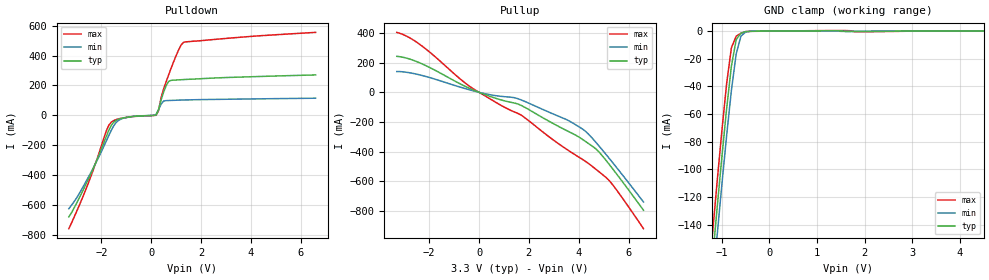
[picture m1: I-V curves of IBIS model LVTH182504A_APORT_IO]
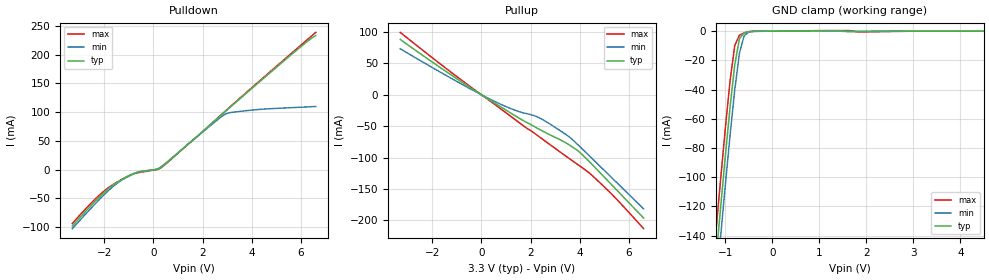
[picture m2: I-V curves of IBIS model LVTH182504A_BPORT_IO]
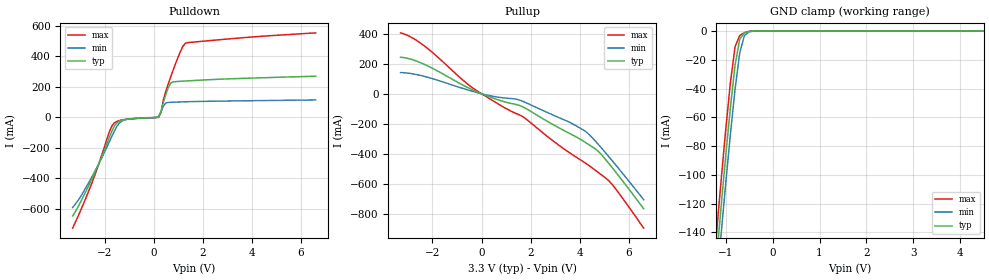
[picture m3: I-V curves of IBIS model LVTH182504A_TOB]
|   TEXAS INSTRUMENTS INCORPORATED
|   Standard Linear and Logic
|   IBIS Model of SN74LVTH182504A
|   3.3V ABT SCAN TEST DEVICES WITH 20-BIT UNIVERSAL BUS TRANSCEIVERS
[IBIS Ver]   2.1
[Comment char]   |_char
[File Name]   sn74lvth182504a.ibs
[File Rev]   1.2   | from silicon model only
[Date]   01/31/2001
[Source]   Silicon-level SPICE model at Texas Instruments (ALEY)
[Notes]
   3.3-V ABT SCAN TEST DEVICES WITH 20-BIT UNIVERSAL BUS TRANSCEIVERS
   !! SN74LVTH182504A is available and preferred vs SN74LVT182504 !!
   Release 1.0) 97104 ALEY
   Release 1.1) 97212 ALEY (based on process model updates)
   Release 1.2) 97215 ALEY - fixed load for ramp (rising) measurement
   includes all available commercial packages:
   PM=64TQFP (no-coupling model)
   - This file may be incomplete or may not be fully compliant
   with the IBIS specification. It will be replaced with a
   version that is IBIS Revision 3.2 compliant and is complete
   and accurate. Please email all questions and comments to
   sllibis@ti.com.
|   -For Questions or Comments please mailto:sllibis@ti.com
|  [Disclaimer]
|*   Property of Texas Instruments Incorporated.  Unauthorized   *
|*   reproduction and/or distribution is strictly prohibited.   *
|*   This product is protected under copyright law.   *
|*   Created 1995, (C) Copyright 1995, Texas Instruments Inc.,   *
|*   All Rights Reserved   *
|*   UNLESS THERE IS A SIGNED, WRITTEN AGREEMENT TO THE   *
|*   CONTRARY, TEXAS INSTRUMENTS ("TI") IS PROVIDING THE SPICE   *
|*   MODELS "AS IS" AND WITHOUT ANY WARRANTY, EXPRESSED OR   *
|*   IMPLIED.  TI assumes no liability for:   *
|*   1) the accuracy of the IBIS models provided to your   *
|*   company;   *
|*   2) the proper functioning of these IBIS models in your   *
|*   design or for any resulting applications; or   *
|*   3) infringement of patents, copyrights or intellectual   *
|*   property rights resulting from your use of these   *
|*   IBIS models.   *
|*   TI provides IBIS Models as a service to our customers.   *
|*   You and your company shall not distribute, sell or give   *
|*   these models to anyone else without prior written   *
|*   permission from TI.   *
|*   TI reserves the right to make changes to our products or   *
|*   to discontinue any semiconductor product or service   *
|*   without notice, and advises our customers to obtain the   *
|*   latest version of relevant information to verify, before   *
|*   placing orders, that the information being relied on is   *
|*   current.   *
|*   Please be aware that your receipt and use of the IBIS   *
|*   information provided shall serve as acceptance of these   *
|*   terms and conditions.  If you do not accept these terms,   *
|*   you should return or destroy the IBIS models and any   *
|*   other accompanying information immediately.   *
[Component]   SN74LVTH182504APM
[Manufacturer]  Texas Instruments
[Package]
|   typ   min   max
R_pkg   0.03   0.027   0.034
L_pkg   2.066nH   1.969nH   2.225nH
C_pkg   0.104pF   0.075pF   0.188pF
[Pin]   signal_name  model_name   R_pin   L_pin   C_pin
1   A4   LVTH182504A_APORT_IO   0.03   2.212nH   0.188pF
2   A5   LVTH182504A_APORT_IO   0.029   2.132nH   0.114pF
3   A6   LVTH182504A_APORT_IO   0.03   2.093nH   0.099pF
4   GND   GND   0.03   2.08nH   0.106pF
5   A7   LVTH182504A_APORT_IO   0.032   2.05nH   0.087pF
6   A8   LVTH182504A_APORT_IO   0.032   2.015nH   0.08pF
7   A9   LVTH182504A_APORT_IO   0.033   2.007nH   0.077pF
8   A10   LVTH182504A_APORT_IO   0.032   1.99nH   0.08pF
9   VCC   POWER   0.033   2.074nH   0.09pF
10   A11   LVTH182504A_APORT_IO   0.032   1.995nH   0.075pF
11   A12   LVTH182504A_APORT_IO   0.032   2.025nH   0.08pF
12   A13   LVTH182504A_APORT_IO   0.031   2.033nH   0.085pF
13   GND   GND   0.03   2.093nH   0.105pF
14   A14   LVTH182504A_APORT_IO   0.031   2.142nH   0.1pF
15   A15   LVTH182504A_APORT_IO   0.03   2.166nH   0.114pF
16   A16   LVTH182504A_APORT_IO   0.029   2.225nH   0.188pF
17   A17   LVTH182504A_APORT_IO   0.03   2.213nH   0.188pF
18   A18   LVTH182504A_APORT_IO   0.031   2.161nH   0.114pF
19   A19   LVTH182504A_APORT_IO   0.032   2.142nH   0.1pF
20   GND   GND   0.031   2.106nH   0.105pF
21   A20   LVTH182504A_APORT_IO   0.032   2.054nH   0.085pF
22   NCLKENAB  LVTH182504A_INC   0.032   2.017nH   0.077pF
23   CLKAB   LVTH182504A_INC   0.033   2.065nH   0.079pF
24   TDI   LVTH182504A_INU   0.034   2.087nH   0.084pF
25   VCC   POWER   0.032   2.049nH   0.086pF
26   TCK   LVTH182504A_INT   0.032   1.989nH   0.075pF
27   LEAB   LVTH182504A_INC   0.032   2.014nH   0.079pF
28   NOEAB   LVTH182504A_INU   0.032   2.049nH   0.086pF
29   GND   GND   0.03   2.073nH   0.105pF
30   B20   LVTH182504A_BPORT_IO   0.03   2.097nH   0.099pF
31   B19   LVTH182504A_BPORT_IO   0.031   2.142nH   0.114pF
32   B18   LVTH182504A_BPORT_IO   0.028   2.178nH   0.187pF
33   B17   LVTH182504A_BPORT_IO   0.028   2.167nH   0.187pF
34   B16   LVTH182504A_BPORT_IO   0.027   2.082nH   0.112pF
35   B15   LVTH182504A_BPORT_IO   0.029   2.08nH   0.099pF
36   GND   GND   0.029   2.064nH   0.105pF
37   B14   LVTH182504A_BPORT_IO   0.029   2.008nH   0.085pF
38   B13   LVTH182504A_BPORT_IO   0.03   1.98nH   0.079pF
39   B12   LVTH182504A_BPORT_IO   0.031   1.981nH   0.077pF
40   B11   LVTH182504A_BPORT_IO   0.031   1.976nH   0.08pF
41   VCC   POWER   0.033   2.005nH   0.081pF
42   B10   LVTH182504A_BPORT_IO   0.031   1.97nH   0.076pF
43   B9   LVTH182504A_BPORT_IO   0.031   1.996nH   0.08pF
44   B8   LVTH182504A_BPORT_IO   0.031   2.03nH   0.086pF
45   GND   GND   0.03   2.072nH   0.105pF
46   B7   LVTH182504A_BPORT_IO   0.03   2.102nH   0.1pF
47   B6   LVTH182504A_BPORT_IO   0.029   2.11nH   0.113pF
48   B5   LVTH182504A_BPORT_IO   0.028   2.155nH   0.186pF
49   B4   LVTH182504A_BPORT_IO   0.028   2.157nH   0.186pF
50   B3   LVTH182504A_BPORT_IO   0.028   2.09nH   0.112pF
51   B2   LVTH182504A_BPORT_IO   0.028   2.078nH   0.099pF
52   GND   GND   0.029   2.047nH   0.105pF
53   B1   LVTH182504A_BPORT_IO   0.028   1.996nH   0.085pF
54   NCLKENBA  LVTH182504A_INC   0.029   1.969nH   0.079pF
55   CLKBA   LVTH182504A_INC   0.031   1.97nH   0.077pF
56   TMS   LVTH182504A_INU   0.031   1.975nH   0.08pF
57   VCC   POWER   0.032   1.985nH   0.08pF
58   TDO   LVTH182504A_TOB   0.031   1.98nH   0.077pF
59   LEBA   LVTH182504A_INC   0.03   1.987nH   0.08pF
60   NOEBA   LVTH182504A_INU   0.03   2.022nH   0.086pF
61   GND   GND   0.029   2.068nH   0.105pF
62   A1   LVTH182504A_APORT_IO   0.03   2.086nH   0.099pF
63   A2   LVTH182504A_APORT_IO   0.029   2.117nH   0.113pF
64   A3   LVTH182504A_APORT_IO   0.029   2.167nH   0.186pF
| Models and submodels in the file (6): LVTH182504A_APORT_IO (I/O), LVTH182504A_BPORT_IO (I/O), LVTH182504A_TOB (3-state), LVTH182504A_INC (Input), LVTH182504A_INT (Input), LVTH182504A_INU (Input)
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[Model]   LVTH182504A_APORT_IO
| high-drive I/O buffer with bus-hold
| ibuf.lvta (97212 ALEY)
| tob.lvta  (97212 ALEY)
| pad.lvta  (97212 ALEY)
| Signals   A1..A20
Model_type  I/O
Polarity   Non-Inverting
Enable   Active-Low
Vinl = 0.8V
Vinh = 2.0V
Vmeas= 1.5V
Cref = 50pf
Rref = 500
Vref = 0V
| variable   typ   min   max
C_comp   10p   NA   NA
[Temperature Range]   50   100   0
[Voltage range]   3.3   3   3.6
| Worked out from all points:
|   slope of the pulldown table from 0 to 0.495 V, typ, clamps not added: 3.25 ohm
|   slope of the pullup table from 0 to 0.495 V, typ, clamps not added: 16.2 ohm
|   GND clamp passes 1 mA (typ) near -0.56 V on its own axis
|Process range|   weak   strong
[pullup]
|   50C:3.3V:   100C:3V:weak   0C:3.6V:strong
|   Voltage   I(typ)   I(min)   I(max)
-3.3V     242.7mA    140.2mA    404.2mA
-2.8V     225.4mA    132.2mA    369.3mA
-2.3V     192.9mA    114.1mA    313.8mA
-300mV    20.86mA    13.18mA    31.49mA
700mV     -41.94mA   -23.2mA    -70.26mA
1.5V      -75.64mA   -39.93mA   -138.1mA
1.8V      -97.86mA   -58.74mA   -166.6mA
3.6V      -265.2mA   -191.6mA   -393.7mA
4.3V      -334.7mA   -267.1mA   -469.1mA
4.7V      -383.4mA   -339.3mA   -520.3mA
5.2V      -480.9mA   -440.4mA   -590.8mA
6.6V      -795.3mA   -739.8mA   -919.7mA
[pulldown]
|   50C:3.3V:   100C:3V:weak   0C:3.6V:strong
|   Voltage   I(typ)   I(min)   I(max)
-3.3V     -677.8mA   -623.8mA   -757mA
-2.5V     -420.1mA   -407.9mA   -444.4mA
-1.8V     -141.6mA   -172.1mA   -104.6mA
-1.6V     -67.02mA   -100.3mA   -45.51mA
-1.4V     -32.5mA    -46.74mA   -27.93mA
200mV     2.567mA    6.67mA     823.3uA
300mV     39.57mA    39.07mA    32.13mA
500mV     154.4mA    95.69mA    175mA
700mV     226.4mA    99.55mA    269.2mA
1.1V      237.5mA    101.9mA    436.1mA
1.3V      239.4mA    103mA      488.3mA
6.6V      270.5mA    114.9mA    554.8mA
[gnd_clamp]
|   50C:3.3V:   100C:3V:weak   0C:3.6V:strong
|   Voltage   I(typ)   I(min)   I(max)
-3.3V     -1.549A    -1.512A    -1.612A
-1.2V     -166.4mA   -186.3mA   -147.8mA
-1.1V     -128.1mA   -148mA     -109.1mA
-1V       -91.01mA   -111mA     -72.06mA
-900mV    -56mA      -75.56mA   -37.94mA
-800mV    -25.34mA   -42.9mA    -12mA
-700mV    -6.279mA   -16.54mA   -3.704mA
-600mV    -1.455mA   -3.641mA   -1.512mA
-500mV    -329uA     -657.6uA   -358.3uA
-300mV    -77.95uA   -53.31uA   -119.1uA
1.4V      233.8uA    101uA      404.8uA
6.6V      11.17nA    12.21nA    10.92nA
[ramp]
| variable   typ   min   max
dV/dt_r   1.5089E+00/4.8115E-10  1.1420E+00/1.4491E-09  1.7783E+00/2.2391E-10
dV/dt_f   1.7910E+00/8.5545E-10  1.6177E+00/2.2914E-09  1.9765E+00/4.1736E-10
[Model]   LVTH182504A_BPORT_IO
| high-drive I/O buffer with bus-hold
| ibuf.lvta (97212 ALEY)
| t25.lvta  (97212 ALEY)
| pad.lvta  (97212 ALEY)
| Signals   B1..B20
Model_type  I/O
Polarity   Non-Inverting
Enable   Active-Low
Vinl = 0.8V
Vinh = 2.0V
Vmeas= 1.5V
Cref = 50pf
Rref = 500
Vref = 0V
| variable   typ   min   max
C_comp   10p   NA   NA
[Temperature Range]   50   100   0
[Voltage range]   3.3   3   3.6
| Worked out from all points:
|   slope of the pulldown table from 0 to 0.495 V, typ, clamps not added: 45.3 ohm
|   slope of the pullup table from 0 to 0.495 V, typ, clamps not added: 40.7 ohm
|   GND clamp passes 1 mA (typ) near -0.58 V on its own axis
|Process range|   weak   strong
[pullup]
|   50C:3.3V:   100C:3V:weak   0C:3.6V:strong
|   Voltage   I(typ)   I(min)   I(max)
-3.3V     87.93mA    73.1mA     99.21mA
-1.6V     41.29mA    34.42mA    46.83mA
200mV     -4.944mA   -4.077mA   -5.666mA
1.3V      -31.73mA   -23.61mA   -37.44mA
2.3V      -53.86mA   -35.71mA   -65.38mA
3.2V      -71.57mA   -57.06mA   -91.07mA
3.6V      -80.55mA   -67.91mA   -102.3mA
3.9V      -88.5mA    -78.65mA   -110.6mA
4.5V      -110.9mA   -101.4mA   -128.3mA
5.4V      -147.4mA   -135.8mA   -162.2mA
6.6V      -196.3mA   -181.6mA   -213.2mA
[pulldown]
|   50C:3.3V:   100C:3V:weak   0C:3.6V:strong
|   Voltage   I(typ)   I(min)   I(max)
-3.3V     -98.29mA   -102.9mA   -93.91mA
-2.3V     -52.13mA   -56.52mA   -48.52mA
-1.9V     -35.93mA   -39.45mA   -33.8mA
-1.5V     -22.87mA   -24.62mA   -22.42mA
-700mV    -5.307mA   -5.472mA   -6.239mA
100mV     25.12uA    283.8uA    -376.2uA
300mV     3.666mA    4.577mA    2.833mA
2.9V      100.2mA    95.86mA    100.8mA
3.1V      107.6mA    98.94mA    108.5mA
4.2V      148.5mA    104.2mA    149.9mA
6V        214mA      108.5mA    216.5mA
6.6V      233.1mA    109.7mA    238.6mA
[gnd_clamp]
|   50C:3.3V:   100C:3V:weak   0C:3.6V:strong
|   Voltage   I(typ)   I(min)   I(max)
-3.3V     -969.6mA   -991mA     -949.1mA
-1.2V     -156.2mA   -176mA     -137mA
-1.1V     -120.2mA   -140.1mA   -101mA
-1V       -85.23mA   -105mA     -66.15mA
-900mV    -52mA      -71.24mA   -33.96mA
-800mV    -22.87mA   -40.05mA   -9.759mA
-700mV    -5.117mA   -14.95mA   -2.748mA
-600mV    -1.165mA   -3.046mA   -1.228mA
-500mV    -309.2uA   -581.3uA   -349.3uA
-300mV    -77.95uA   -53.3uA    -119.1uA
1.4V      233.8uA    101uA      404.8uA
6.6V      11.17nA    12.21nA    10.92nA
[ramp]
| variable   typ   min   max
dV/dt_r   1.0791E+00/4.8409E-10  8.6453E-01/1.4920E-09  1.2563E+00/2.4887E-10
dV/dt_f   1.2133E+00/7.4384E-10  1.1004E+00/1.8193E-09  1.3392E+00/3.7318E-10
[Model]   LVTH182504A_TOB
| three-state output buffer
| tob.lvta (97212 ALEY)
| pad.lvta (97212 ALEY)
| Signals   TDO
Model_type  3-state
Polarity   Non-Inverting
Enable   Active-Low
Vinl = 0.8V
Vinh = 2.0V
Vmeas= 1.5V
Cref = 50pf
Rref = 500
Vref = 0V
| variable   typ   min   max
C_comp   8p   NA   NA
[Temperature Range]   50   100   0
[Voltage range]   3.3   3   3.6
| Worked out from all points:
|   slope of the pulldown table from 0 to 0.495 V, typ, clamps not added: 3.25 ohm
|   slope of the pullup table from 0 to 0.495 V, typ, clamps not added: 16.2 ohm
|   GND clamp passes 1 mA (typ) near -0.58 V on its own axis
|Process range|   weak   strong
[pullup]
|   50C:3.3V:   100C:3V:weak   0C:3.6V:strong
|   Voltage   I(typ)   I(min)   I(max)
-3.3V     242.7mA    140.2mA    404.2mA
-2.8V     225.4mA    132.2mA    369.3mA
-2.3V     192.9mA    114.1mA    313.8mA
-300mV    20.86mA    13.18mA    31.49mA
700mV     -41.88mA   -23.15mA   -70.19mA
1.5V      -75.36mA   -39.76mA   -137.7mA
1.8V      -97.58mA   -58.87mA   -166.1mA
3.6V      -265.1mA   -191mA     -393.7mA
4.3V      -331mA     -259mA     -468.4mA
4.7V      -375mA     -326.3mA   -516.3mA
5.2V      -466.4mA   -421.4mA   -580.8mA
6.6V      -763.6mA   -703.5mA   -892.5mA
[pulldown]
|   50C:3.3V:   100C:3V:weak   0C:3.6V:strong
|   Voltage   I(typ)   I(min)   I(max)
-3.3V     -646.1mA   -591.2mA   -726.1mA
-2.5V     -398.2mA   -385.2mA   -423.3mA
-1.8V     -128.3mA   -158mA     -92.21mA
-1.6V     -56.18mA   -88.6mA    -35.51mA
-1.4V     -24.07mA   -37.43mA   -20.33mA
200mV     2.519mA    6.639mA    748.6uA
300mV     39.5mA     39.03mA    32.02mA
500mV     154.3mA    95.61mA    174.8mA
700mV     226.2mA    99.46mA    268.9mA
1.1V      237.3mA    101.8mA    435.7mA
1.3V      239.2mA    102.8mA    487.9mA
6.6V      270.5mA    114.9mA    554.8mA
[gnd_clamp]
|   50C:3.3V:   100C:3V:weak   0C:3.6V:strong
|   Voltage   I(typ)   I(min)   I(max)
-3.3V     -1.517A    -1.479A    -1.581A
-1.2V     -160.3mA   -179.4mA   -142.5mA
-1.1V     -123.2mA   -142.2mA   -105mA
-1V       -87.28mA   -106.4mA   -69.11mA
-900mV    -53.39mA   -72.1mA    -36.02mA
-800mV    -23.77mA   -40.53mA   -10.91mA
-700mV    -5.596mA   -15.18mA   -3.038mA
-600mV    -1.236mA   -3.105mA   -1.085mA
-500mV    -194.2uA   -518.2uA   -118.5uA
-400mV    -8.285uA   -43.13uA   -1.218uA
6.6V      7.886nA    8.661nA    7.714nA
[ramp]
| variable   typ   min   max
dV/dt_r   1.5081E+00/4.7366E-10  1.1387E+00/1.4512E-09  1.7781E+00/2.1597E-10
dV/dt_f   1.7910E+00/8.4858E-10  1.6182E+00/2.2837E-09  1.9768E+00/4.0623E-10
